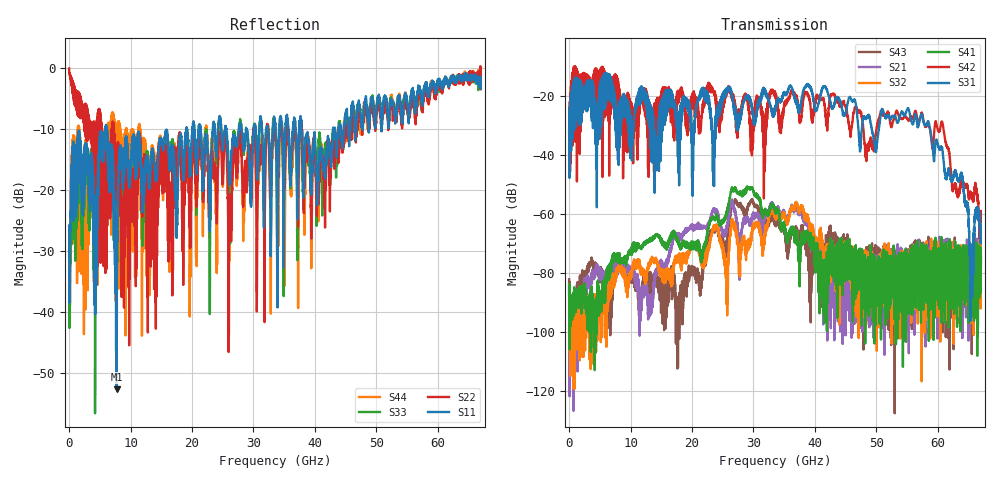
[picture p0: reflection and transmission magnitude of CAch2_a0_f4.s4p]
!Agilent Technologies,N5247A,US51170199,A.09.90.13
!Agilent N5247A: A.09.90.13
!Date: Thursday, October 18, 2018 11:33:57
!Correction: S11(Full 4 Port(1,2,3,4))
!S12(Full 4 Port(1,2,3,4))
!S13(Full 4 Port(1,2,3,4))
!S14(Full 4 Port(1,2,3,4))
!S21(Full 4 Port(1,2,3,4))
!S22(Full 4 Port(1,2,3,4))
!S23(Full 4 Port(1,2,3,4))
!S24(Full 4 Port(1,2,3,4))
!S31(Full 4 Port(1,2,3,4))
!S32(Full 4 Port(1,2,3,4))
!S33(Full 4 Port(1,2,3,4))
!S34(Full 4 Port(1,2,3,4))
!S41(Full 4 Port(1,2,3,4))
!S42(Full 4 Port(1,2,3,4))
!S43(Full 4 Port(1,2,3,4))
!S44(Full 4 Port(1,2,3,4))
!S4P File: Measurements: <S11,S12,S13,S14>,
!<S21,S22,S23,S24>,
!<S31,S32,S33,S34>,
!<S41,S42,S43,S44>:
# Hz S  dB  R 50
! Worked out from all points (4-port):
!   6701 points, 10 MHz to 67 GHz, reference 50 ohm
!   strongest paths, dB at 10 MHz, 16.76 GHz, 33.51 GHz, 50.25 GHz, 67 GHz:
!     S31: -33.5, -23.3, -23.9, -33.6, -69.3
!     S42: -32.1, -27.2, -18.7, -28.6, -60.0
!     S41: -84.0, -66.5, -59.0, -80.9, -77.6
!     S32: -90.6, -80.2, -61.1, -83.6, -73.6
!     S21: -85.9, -69.7, -60.4, -80.1, -75.0
!     S43: -82.2, -85.6, -62.5, -73.8, -75.0
!   lowest |S11| = -52.7 dB at 7.759 GHz (marker M1), VSWR 1.00, Z = 49.8 - j0.111 ohm
!   |S11| at or under -10 dB: start of sweep to 5.878 GHz; 6.109 GHz to 19.04 GHz (12.93 GHz wide, 103 % of centre); 37.83 GHz to 42.99 GHz (5.162 GHz wide, 12.8 % of centre)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
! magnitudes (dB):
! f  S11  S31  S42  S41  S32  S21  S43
! 10 MHz  -25.9  -33.5  -32.1  -84.0  -90.6  -85.9  -82.2
! 5.979 GHz  -9.6  -12.4  -12.9  -84.7  -90.4  -83.5  -84.9
! 7.759 GHz  -52.7  -29.5  -21.1  -73.6  -79.1  -77.9  -77.6
! 21.42 GHz  -10.4  -18.3  -30.7  -75.6  -75.6  -65.0  -87.5
! 29.34 GHz  -15.6  -21.1  -25.8  -51.3  -70.5  -62.9  -56.6
! 55.11 GHz  -6.6  -24.2  -28.1  -74.0  -90.5  -78.5  -77.7
! 67 GHz  -3.4  -69.3  -60.0  -77.6  -73.6  -75.0  -75.0
